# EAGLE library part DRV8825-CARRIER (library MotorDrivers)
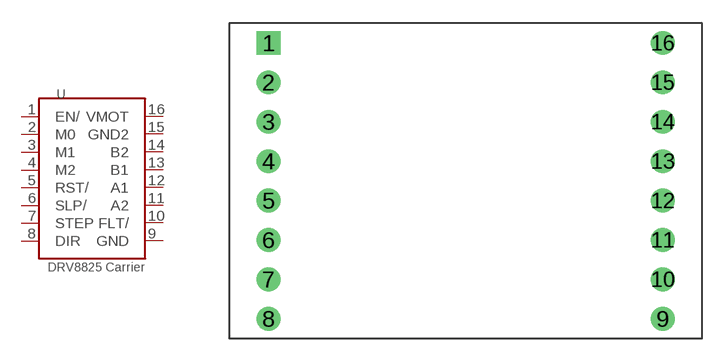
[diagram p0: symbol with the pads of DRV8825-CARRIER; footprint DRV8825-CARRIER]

Designator prefix U

## DRV8825-CARRIER  [DRV8825-CARRIER]
1  EN/
2  M0
3  M1
4  M2
5  RST/
6  SLP/
7  STEP
8  DIR
9  GND
10  FLT/
11  A2
12  A1
13  B1
14  B2
15  GND2
16  VMOT

## Footprint DRV8825-CARRIER (pad centres in mm)
drill 1.016 square: 1 -12.7,8.89
drill 1.016: 2 -12.7,6.35; 3 -12.7,3.81; 4 -12.7,1.27; 5 -12.7,-1.27; 6 -12.7,-3.81; 7 -12.7,-6.35; 8 -12.7,-8.89; 9 12.7,-8.89; 10 12.7,-6.35; 11 12.7,-3.81; 12 12.7,-1.27; 13 12.7,1.27; 14 12.7,3.81; 15 12.7,6.35; 16 12.7,8.89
